VAR_GLOBAL
	//输入
	limit_switch_up  AT%I*:BOOL;               //上限位
	limit_switch_down AT%I*:BOOL;              //下限位
	//输出
	solenoid_valve_up AT%Q*:BOOL;              //上行电磁阀
	solenoid_valve_down AT%Q*:BOOL;            //下行电磁阀
END_VAR
